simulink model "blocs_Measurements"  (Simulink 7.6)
settings: Solver=ode15s  StartTime=0.0  StopTime=0.1  RelTol=1e-3
InitFcn:
  | clc
  | close all
  | clear all
  | Ts=50e-6;
StopFcn:
  | load Somme_sinus_filtre.mat
  | plot(x(1,:),x(2,:),x(1,:),x(3,:),x(1,:),x(4,:))
  | grid
  | title('sinusoïde 60 Hz, somme et sortie du filtre')
  | xlabel('temps')
  | 
  | figure
  | load Fourier_RMS_Mean.mat
  | plot(y(1,:),y(2,:),y(1,:),y(3,:),y(1,:),y(4,:))
  | grid
  | title('Fourier, RMS et Mean')
  | xlabel('temps')
libraries: powerlib x6, powerlib_extras x4

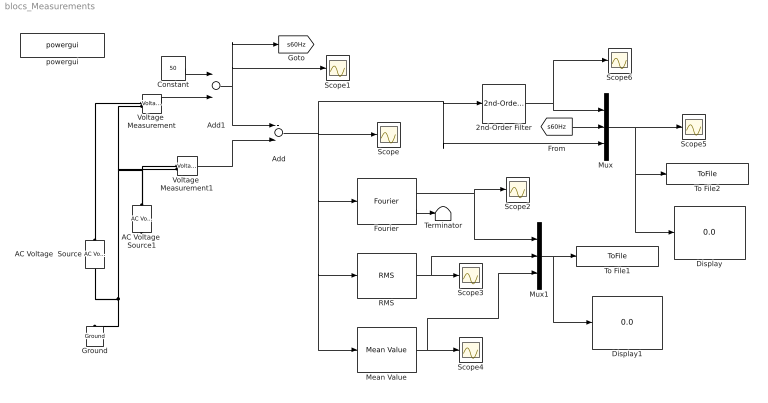
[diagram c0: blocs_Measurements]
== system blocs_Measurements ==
  2nd-Order Filter : powerlib_extras/Control  Blocks/2nd-Order Filter  DialogController=POWERSYS.PowerSysDialog  SystemSampleTime=-1  FilterType=Lowpass  Fo=70  Zeta=0.707  Initialize=off  Vac_Init=[1 45 60]  Vdc_Init=-0.5  PlotResponse=off  param1=[1 500 1]
  AC Voltage  Source : powerlib/Electrical Sources/AC Voltage Source  DialogController=POWERSYS.PowerSysDialog  SystemSampleTime=-1  Amplitude=100  Phase=0  Frequency=60  SampleTime=0  Measurements=None
  AC Voltage  Source1 : powerlib/Electrical Sources/AC Voltage Source  DialogController=POWERSYS.PowerSysDialog  SystemSampleTime=-1  Amplitude=50  Phase=0  Frequency=120  SampleTime=0  Measurements=None
  Add : Sum
  Add1 : Sum
  Constant : Constant  Value=50
  Display : Display
  Display1 : Display
  Fourier : powerlib_extras/Measurements/Fourier  DialogController=POWERSYS.PowerSysDialog  SystemSampleTime=-1  f1=60  n=1
  Ground : powerlib/Elements/Ground  DialogController=POWERSYS.PowerSysDialog  PhysicalDomain=powersysdomain  SubClassName=unknown  LeftPortType=p1  RightPortType=p1  LConnTagsString=a
  Mean Value : powerlib_extras/Measurements/Mean Value  DialogController=POWERSYS.PowerSysDialog  SystemSampleTime=-1  Period=1/60
  Mux : Mux  Inputs=3
  Mux1 : Mux  Inputs=3
  RMS : powerlib_extras/Measurements/RMS  DialogController=POWERSYS.PowerSysDialog  SystemSampleTime=-1  f1=60
  Scope{,1..6} (7 alike) : Scope
  Terminator : Terminator
  To File1 : ToFile  Filename=Fourier_RMS_Mean  MatrixName=y
  To File2 : ToFile  Filename=Somme_sinus_filtre  MatrixName=x
  Voltage  Measurement : powerlib/Measurements/Voltage Measurement  DialogController=POWERSYS.PowerSysDialog  SystemSampleTime=-1  PhasorSimulation=off  OutputType=Complex  PSBequivalent=0
  Voltage  Measurement1 : powerlib/Measurements/Voltage Measurement  DialogController=POWERSYS.PowerSysDialog  SystemSampleTime=-1  PhasorSimulation=off  OutputType=Complex  PSBequivalent=0
  powergui : powerlib/powergui  Priority=1  SystemSampleTime=-1  SimulationMode=Continuous  SampleTime=Ts  frequency=60  SPID=off  DisableSnubberDevices=off  DisableRonSwitches=off  DisableVfSwitches=off  SwTol=0  Interpol=off  frequencyindice=60  echomessages=off  HookPort=off  DisplayEquations=off  FunctionMessages=off  EnableUseOfTLC=off  x0status=blocks  RestoreLinks=warning  ResistiveCurrentMeasurement=off  Ylog=off  Xlog=on  ShowGrid=off  save=off  variable=ZData  ZoomFFT=off  StartTime=0.0  cycles=1  DisplayStyle=1  fundamental=60  FreqAxis=off  MaxFrequency=1000  frequencyindicesteady=1  display=off  methode=off
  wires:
  Voltage  Measurement1/1 -> Add/2
  Add/1 -> Scope/1, Fourier/1, Mean Value/1, RMS/1, 2nd-Order Filter/1, Mux/3
  Voltage  Measurement/1 -> Add1/2
  Constant/1 -> Add1/1
  Add1/1 -> Add/1, Scope1/1, [s60Hz]
  Fourier/1 -> Scope2/1, Mux1/1
  RMS/1 -> Scope3/1, Mux1/2
  Mean Value/1 -> Scope4/1, Mux1/3
  2nd-Order Filter/1 -> Mux/1, Scope6/1
  Mux/1 -> Scope5/1, To File2/1, Display/1
  [s60Hz] -> Mux/2
  Mux1/1 -> To File1/1, Display1/1
  Fourier/2 -> Terminator/1
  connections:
  AC Voltage  Source/LConn1 -- Ground/LConn1 -- AC Voltage  Source1/LConn1 -- Voltage  Measurement1/LConn2 -- Voltage  Measurement/LConn2
  AC Voltage  Source/RConn1 -- Voltage  Measurement/LConn1
  AC Voltage  Source1/RConn1 -- Voltage  Measurement1/LConn1
